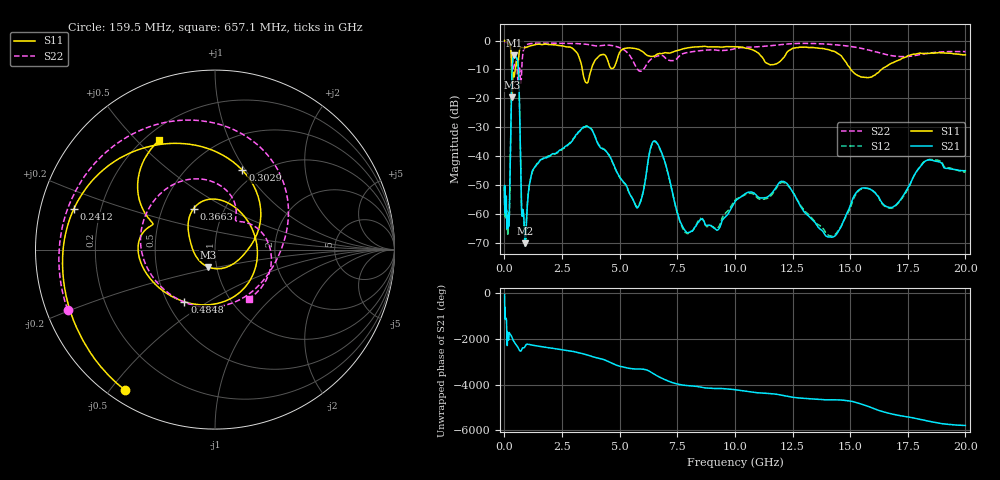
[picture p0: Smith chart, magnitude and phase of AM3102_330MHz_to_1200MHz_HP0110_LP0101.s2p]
! Date/Time: Tue, Sep 11, 2018 5:14 PM
! Network Analyzer: Agilent Technologies E8362B Rev: A.07.50.63
! Sweep from 0.010 to 20.000 GHz, 1601 Points, Sweep Type: LOG
! Power Supply: 4.949 V, 0.001 A
# Hz S DB R 50
!freq MagS11 AngS11 MagS21 AngS21 MagS12 AngS12 MagS22 AngS22
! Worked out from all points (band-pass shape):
!   1601 points, 10 MHz to 20 GHz, reference 50 ohm
!   highest |S21| = -5.08 dB at 434.6 MHz (marker M1); lowest = -70.1 dB at 907.7 MHz (marker M2)
!   |S21| within 3 dB of the highest: 346.4 MHz to 592 MHz (245.6 MHz wide, 52.3 % of centre)
!   lowest |S11| = -19.6 dB at 337.9 MHz (marker M3), VSWR 1.23, Z = 45.6 - j9 ohm
!   |S11| at or under -10 dB: 314.8 MHz to 475.2 MHz (160.4 MHz wide, 40.6 % of centre); 3.379 GHz to 3.771 GHz (392 MHz wide, 11 % of centre); 15.03 GHz to 16.37 GHz (1.34 GHz wide, 8.54 % of centre)
!   |S22| runs from -14.8 to -0.2 dB; largest |S21 - S12| = 0.0093
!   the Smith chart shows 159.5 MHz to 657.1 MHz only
!   S11 on the Smith chart (normalised r, x): 159.5 MHz: 0.05, -0.55; 241.2 MHz: 0.10, +0.14; 302.9 MHz: 0.85, +0.97; 366.3 MHz: 0.71, +0.35; 484.8 MHz: 0.61, -0.40; 657.1 MHz: 0.25, +0.58
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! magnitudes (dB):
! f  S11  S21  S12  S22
! 10 MHz  0.0  -50.9  -50.4  -0.2
! 35.55 MHz  0.0  -57.6  -56.8  -0.4
! 126.4 MHz  -0.4  -62.4  -63.4  -0.9
! 159.5 MHz  -0.6  -63.1  -65.0  -1.0
! 241.2 MHz  -1.7  -49.4  -49.9  -1.8
! 302.9 MHz  -6.6  -19.9  -20.0  -4.0
! 337.9 MHz  -19.6  -9.3  -9.3  -8.3
! 366.3 MHz  -11.8  -6.5  -6.6  -10.1
! 434.6 MHz  -12.2  -5.1  -5.1  -8.2
! 447.2 MHz  -11.5  -5.1  -5.1  -7.8
! 484.8 MHz  -9.5  -5.3  -5.4  -7.3
! 657.1 MHz  -3.3  -22.5  -22.6  -9.6
! 750.6 MHz  -2.4  -59.2  -58.8  -10.3
! 907.7 MHz  -2.5  -70.1  -71.2  -1.9
! 1.59 GHz  -1.4  -41.2  -41.2  -0.9
! 3.634 GHz  -14.2  -29.9  -29.6  -1.4
! 5.652 GHz  -2.7  -56.4  -56.2  -8.2
! 6.58 GHz  -5.0  -35.0  -35.2  -5.5
! 7.92 GHz  -2.6  -66.6  -66.8  -4.2
! 12.09 GHz  -6.2  -48.8  -49.1  -1.3
! 14.07 GHz  -3.2  -68.0  -67.4  -1.3
! 20 GHz  -5.0  -45.0  -45.6  -3.8
